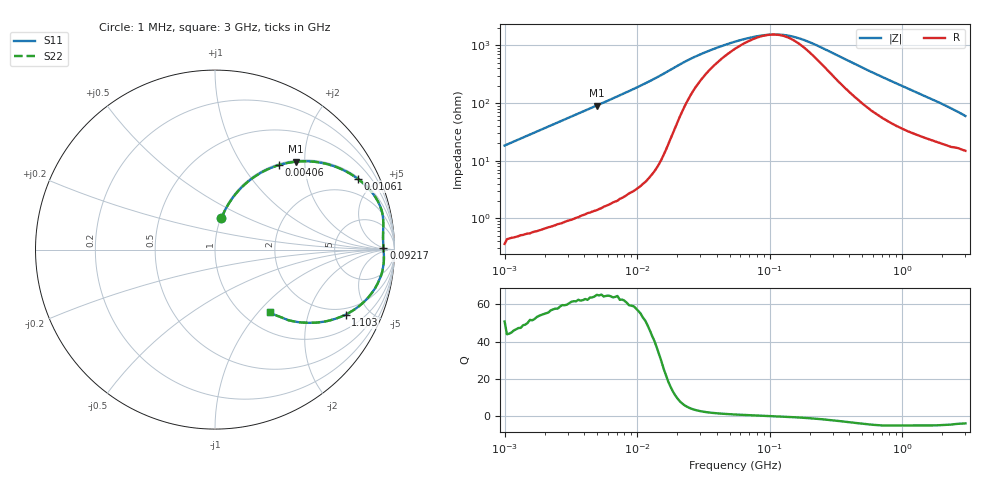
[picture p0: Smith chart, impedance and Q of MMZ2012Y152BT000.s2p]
! S-parameter Generated by TDK Corporation
! Copyright(C) 2016 TDK Corporation.
! All Rights Reserved.
! TDK P/N: MMZ2012Y152BT000 (Chip Beads)
! Property: |Z|=1500¶ at 100MHz
! Size(LxWxT): 2x1.25x0.85mm, 0.079x0.049x0.033inches
! Model Type: s2p (Touchstone File Format Version 1.0)
! Frequency: DC=Yes Start=1MHz Stop=3000MHz 202points Log-sweep
! Note: This model was converted from impedance.
! Model Generated on May. 16, 2016
! Hash(MD5):
! Port Assignments:
!  1 ---@@@--- 2
! Applicable Conditions:
!  Temperature = 25 degC
!  DC Bias Current = 0 A
!  Small Signal Operation
! Terms and conditions regarding TDK Simulation Models
! (1)This simulation model is being provided solely for informational purposes. Please refer to the specifications of the products in terms of detailed characteristics of such products.
! (2)In no event shall TDK Corporation of any of its subsidiaries be liable for any loss or damage arising, directly or indirectly,
!  From any information contained in this simulation model, including, but not limited to loss or damages arising from any inaccuracies, omissions or errors in connection with such information.
! (3)Any and all copyrights on this simulation model are owned by TDK Corporation.
!  Duplication or redistribution of this simulation model without prior written permission from TDK Corporation is prohibited.
! (4)This simulation model is subject to any modification or change without any prior notice.
! (5)Neither TDK Corporation nor any of its subsidiaries shall make any warranty, express or implied,
!  Including but not limited to the correctness, implied warranties of merchantability and fitness for a particular purpose with respect to this simulation models.
! (6)The use of this simulation model shall be deemed to have consented to the terms and conditions hereof.
# MHz S MA R 50
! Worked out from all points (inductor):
!   201 points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, 1 MHz to 3 GHz, reference 50 ohm
!   read as one part in series: L = 2.91 uH near 1.041 MHz
!   highest Q = 64.8 at 4.959 MHz (marker M1), where L = 2.9 uH
!   self-resonance near 103.9 MHz
!   S11 on the Smith chart (normalised r, x): 1 MHz: 1.01, +0.37; 4.06 MHz: 1.02, +1.48; 10.61 MHz: 1.07, +4.00; 92.17 MHz: 31, +5; 1.103 GHz: 1.65, -3.52; 3 GHz: 1.30, -1.15
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1  0.1794 78.5  0.9803 -10.3  0.9803 -10.3  0.1794 78.5
1.553251  0.2714 73.1  0.9572 -15.7  0.9572 -15.7  0.2714 73.1
2.13957  0.3609 67.8  0.9261 -21.2  0.9261 -21.2  0.3609 67.8
2.83156  0.4547 62.0  0.883 -27.0  0.883 -27.0  0.4547 62.0
3.900413  0.574 54.1  0.8097 -35.0  0.8097 -35.0  0.574 54.1
4.059721  0.5894 53.0  0.7985 -36.1  0.7985 -36.1  0.5894 53.0
4.959344  0.6651 47.4  0.7366 -41.7  0.7366 -41.7  0.6651 47.4
7.110411  0.7879 37.1  0.6038 -52.0  0.6038 -52.0  0.7879 37.1
10.61086  0.8879 26.4  0.4442 -62.6  0.4442 -62.6  0.8879 26.4
14.61624  0.937 18.8  0.3223 -69.5  0.3223 -69.5  0.937 18.8
19.34349  0.9539 13.1  0.2275 -71.8  0.2275 -71.8  0.9539 13.1
28.86629  0.9457 7.7  0.1407 -63.5  0.1407 -63.5  0.9457 7.7
54.77226  0.9377 3.0  0.08083 -38.1  0.08083 -38.1  0.9377 3.0
92.16659  0.9384 0.5  0.06226 -8.3  0.06226 -8.3  0.9384 0.5
117.1891  0.9397 -0.6  0.061 8.7  0.061 8.7  0.9397 -0.6
143.1579  0.9411 -1.6  0.06465 23.5  0.06465 23.5  0.9411 -1.6
213.6344  0.943 -4.0  0.08846 47.9  0.08846 47.9  0.943 -4.0
457.0858  0.9277 -11.4  0.204 63.6  0.204 63.6  0.9277 -11.4
800.5644  0.8727 -20.2  0.3509 59.0  0.3509 59.0  0.8727 -20.2
1102.76  0.8126 -26.5  0.454 53.1  0.454 53.1  0.8126 -26.5
1855.641  0.6601 -38.2  0.6308 40.3  0.6308 40.3  0.6601 -38.2
3000  0.4636 -48.9  0.778 26.7  0.778 26.7  0.4636 -48.9
